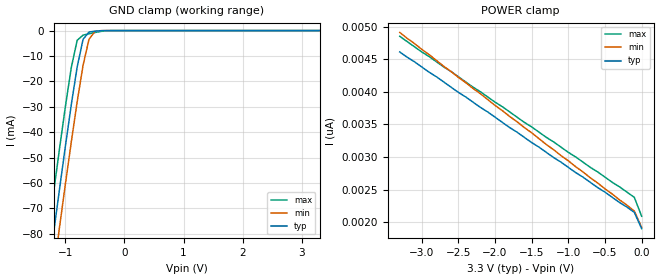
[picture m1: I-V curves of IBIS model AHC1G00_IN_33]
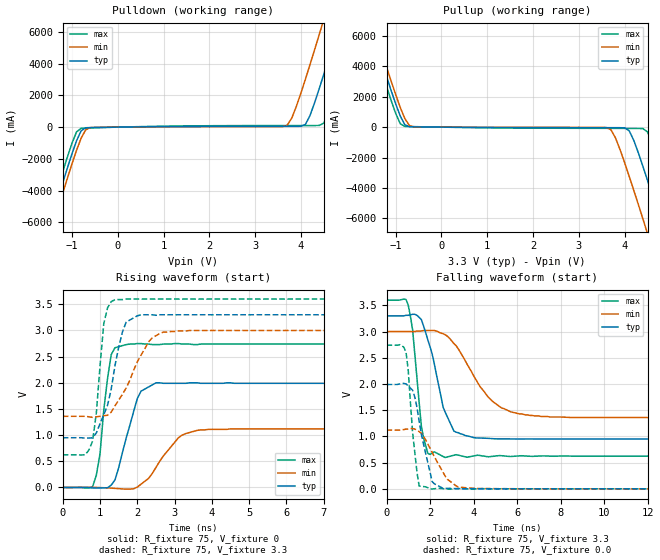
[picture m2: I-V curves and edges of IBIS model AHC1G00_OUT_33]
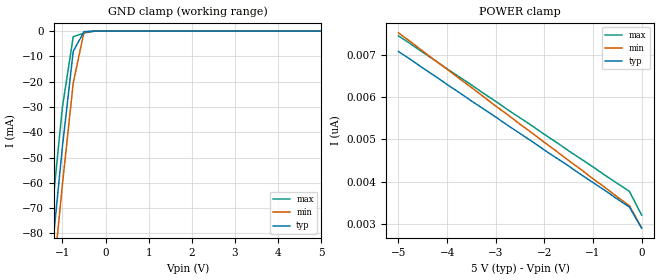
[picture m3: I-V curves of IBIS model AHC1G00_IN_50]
| TEXAS INSTRUMENTS INCORPORATED
| Standard Linear and Logic Group
| IBIS Model of SN74AHC1G00
| SINGLE 2-INPUT POSITIVE-NAND GATE
| SOT 5-pin (DCK) and SOT 5-pin (DBV) Package
[IBIS Ver]   3.2
[Comment Char]  |_char
[File Name]   ahc1g00.ibs
[File Rev]   2.0 J_die
[Date]   May 24, 2000
[Source]   Data created from HSPICE simulations at TI-SLL.
[Notes]   The following is an IBIS list for the AHC1G00.
|   Please contact sllibis@ti.com with questions and
|   comments concerning SLL IBIS models.
[Disclaimer] Property of Texas Instruments Incorporated.  Unauthorized
   reproduction and/or distribution is strictly prohibited.
   This product is protected under copyright law.
   Created 2000, (C) Copyright 2000, Texas Instruments Inc.,
   All Rights Reserved.
   UNLESS THERE IS A SIGNED, WRITTEN AGREEMENT TO THE
   CONTRARY, TEXAS INSTRUMENTS () IS PROVIDING THE IBIS
   MODELS  AND WITHOUT ANY WARRANTY, EXPRESSED OR
   IMPLIED.  TI assumes no liability for:
   1) the accuracy of the IBIS models provided to your
   company;
   2) the proper functioning of these IBIS Models in your
   design or for any resulting applications; or
   3) infringement of patents, copyrights or intellectual
   property rights resulting from your use of these IBIS
   models.
   TI provides IBIS Models as a service to our customers.
   You and your company shall not distribute, sell or give
   these models to anyone else without prior written
   permission from TI.
   TI reserves the right to make changes to our products or
   to discontinue any semiconductor product or service
   without notice, and advises our customers to obtain the
   latest version of relevant information to verify, before
   placing orders, that the information being relied on is
   current.
   Please be aware that your receipt and use of the IBIS
   information provided shall serve as acceptance of these
   terms and conditions.  If you do not accept these terms,
   you should return or destroy the IBIS models and any
   other accompanying information immediately.
|   Component AHC1G00_DCK
[Component]   AHC1G00_DCK
[Manufacturer]  Texas Instruments, Inc.
[Package]
|   typ   min   max
R_pkg   0.020   0.017   0.025
L_pkg   0.998nH   0.881nH   1.069nH
C_pkg   0.146pF   0.118pF   0.205pF
[Pin]   signal_name   model_name   R_pin   L_pin   C_pin
1   A   AHC1G00_IN   0.019   1.069nH   0.162pF
2   B   AHC1G00_IN   0.018   0.881nH   0.121pF
3   GND   GND   0.017   1.031nH   0.205pF
4   Y   AHC1G00_OUT   0.020   0.960nH   0.124pF
5   VCC   POWER   0.025   1.049nH   0.118pF
|   Component AHC1G00_DBV
[Component]   AHC1G00_DBV
[Manufacturer]  Texas Instruments, Inc.
[Package]
|   typ   min   max
R_pkg   0.025   0.021   0.029
L_pkg   1.529nH   1.312nH   1.906nH
C_pkg   0.156pF   0.110pF   0.240pF
[Pin]   signal_name   model_name   R_pin   L_pin   C_pin
1   A   AHC1G00_IN   0.021   1.511nH   0.144pF
2   B   AHC1G00_IN   0.023   1.312nH   0.138pF
3   GND   GND   0.029   1.906nH   0.240pF
4   Y   AHC1G00_OUT   0.026   1.541nH   0.150pF
5   VCC   POWER   0.025   1.374nH   0.110pF
[Model Selector]   AHC1G00_IN
AHC1G00_IN_33   3.3-V Vcc Input Model
AHC1G00_IN_50   5.0-V Vcc Input Model
[Model Selector]   AHC1G00_OUT
AHC1G00_OUT_33   3.3-V Vcc Output Model
AHC1G00_OUT_50   5.0-V Vcc Output Model
| Models and submodels in the file (4): AHC1G00_IN_33 (Input), AHC1G00_OUT_33 (Output), AHC1G00_IN_50 (Input), AHC1G00_OUT_50 (Output)
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|   Model AHC1G00_IN_33
[Model]   AHC1G00_IN_33
Model_type  Input
Polarity   Inverting
Vinl = 0.99
Vinh = 2.31
| variable   typ   min   max
C_comp   1.27pf   0.95pf   1.59pf
[Temperature Range]   25   85   -40
[Voltage Range]   3.3   3.0   3.6
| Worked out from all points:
|   GND clamp passes 1 mA (typ) near -0.61 V on its own axis
[GND Clamp]
|   Voltage   I(typ)   I(min)   I(max)
-3.3V     -460mA     -475mA     -445mA
-1.3V     -97.5mA    -113mA     -81.5mA
-1.2V     -79.9mA    -95mA      -63.9mA
-1.1V     -62.6mA    -77.6mA    -46.7mA
-1V       -45.6mA    -60.5mA    -30mA
-900mV    -29.2mA    -43.9mA    -14.6mA
-800mV    -14.3mA    -28mA      -3.81mA
-700mV    -3.42mA    -13.6mA    -1.78mA
-600mV    -581uA     -3.4mA     -1.25mA
-500mV    -233uA     -353uA     -759uA
-400mV    -58.1uA    -21.9uA    -324uA
3.3V      1.9nA      2.34nA     1.69nA
[POWER Clamp]
|   Voltage   I(typ)   I(min)   I(max)
-3.3V     4.61nA     4.91nA     4.85nA
-3V       4.38nA     4.65nA     4.61nA
-100mV    2.15nA     2.17nA     2.38nA
0V        1.9nA      1.92nA     2.09nA
|   Model AHC1G00_OUT_33
[Model]   AHC1G00_OUT_33
Model_type  Output
Polarity   Inverting
Vmeas = 1.65v
Cref = 15pf
| variable   typ   min   max
C_comp   3.12pf   2.34pf   3.90pf
[Temperature Range]   25   85   -40
[Voltage Range]   3.3   3.0   3.6
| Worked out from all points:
|   slope of the pulldown table from 0 to 0.495 V, typ, clamps not added: 26.1 ohm
|   slope of the pullup table from 0 to 0.495 V, typ, clamps not added: 40.3 ohm
|   rising waveform, R_fixture 75, V_fixture 0: 20-80 % time 450ps typ, 685ps min, 249ps max; typ from 0 V to 1.99 V
|   falling waveform, R_fixture 75, V_fixture 3.3: 20-80 % time 837ps typ, 1.53ns min, 390ps max; typ from 3.3 V to 0.95 V
|   rising waveform, R_fixture 75, V_fixture 3.3: 20-80 % time 435ps typ, 701ps min, 222ps max; typ from 0.95 V to 3.3 V
|   falling waveform, R_fixture 75, V_fixture 0.0: 20-80 % time 576ps typ, 878ps min, 329ps max; typ from 1.99 V to 0 V
[Pulldown]
|   Voltage   I(typ)   I(min)   I(max)
-3.3V     -24A       -24.6A     -23.4A
-1.6V     -7.31A     -7.95A     -6.63A
-1.5V     -6.34A     -6.99A     -5.66A
-1V       -1.69A     -2.33A     -1.02A
-800mV    -234mA     -703mA     -70.7mA
-600mV    -28.4mA    -27.3mA    -48.1mA
3.7V      47.1mA     113mA      100mA
4.1V      173mA      3.03A      101mA
4.4V      2.42A      5.83A      105mA
4.8V      6.17A      9.67A      2.68A
5.2V      10A        13.6A      6.5A
6.6V      23.8A      27.4A      20.3A
[Pullup]
|   Voltage   I(typ)   I(min)   I(max)
-3.3V     23.8A      24.4A      23.2A
-1.6V     7.13A      7.74A      6.5A
-1.5V     6.17A      6.78A      5.53A
-1V       1.53A      2.14A      903mA
-800mV    158mA      559mA      49mA
-600mV    19.5mA     16.8mA     33.4mA
3.7V      -35.9mA    -168mA     -78.9mA
4.1V      -236mA     -3.23A     -83.5mA
4.4V      -2.58A     -6.03A     -95.5mA
4.8V      -6.34A     -9.88A     -2.81A
5.2V      -10.2A     -13.8A     -6.63A
6.6V      -24A       -27.6A     -20.4A
[Ramp]
| variable   typ   min   max
dV/dt_r   1.21E+00/4.52E-10   6.94E-01/6.99E-10   1.65E+00/2.52E-10
dV/dt_f   1.43E+00/7.64E-10   1.00E+00/1.55E-09   1.81E+00/3.63E-10
R_load = 75
[Rising Waveform]
R_fixture = 75
V_fixture = 0
|   Time   V(typ)   V(min)   V(max)
0s        0V         0V         0V
800ps     -8.66mV    1.87mV     14.2mV
1ns       -9.36mV    -2.54mV    650mV
1.1ns     -7.48mV    -5.53mV    1.48V
1.3ns     45.1mV     -12.5mV    2.54V
1.7ns     942mV      -32.5mV    2.73V
2.1ns     1.84V      63mV       2.75V
3.1ns     1.99V      948mV      2.75V
3.9ns     1.99V      1.11V      2.74V
25ns      1.99V      1.12V      2.74V
[Falling Waveform]
R_fixture = 75
V_fixture = 3.3
V_fixture_min = 3.0
V_fixture_max = 3.6
|   Time   V(typ)   V(min)   V(max)
0s        3.3V       3V         3.6V
1ns       3.31V      3V         3.5V
1.2ns     3.33V      3V         3.03V
1.6ns     3.23V      3.01V      1.2V
2ns       2.71V      3.02V      657mV
2.6ns     1.56V      2.96V      617mV
3.1ns     1.1V       2.77V      641mV
4ns       978mV      2.16V      626mV
6.8ns     950mV      1.39V      621mV
25ns      950mV      1.36V      624mV
[Rising Waveform]
R_fixture = 75
V_fixture = 3.3
V_fixture_min = 3.0
V_fixture_max = 3.6
|   Time   V(typ)   V(min)   V(max)
0s        950mV      1.36V      624mV
600ps     944mV      1.36V      624mV
800ps     950mV      1.34V      886mV
900ps     1.04V      1.35V      1.42V
1.1ns     1.39V      1.37V      3.13V
1.4ns     2.33V      1.56V      3.59V
1.7ns     3.16V      1.9V       3.6V
2.3ns     3.3V       2.78V      3.6V
2.7ns     3.3V       2.97V      3.6V
25ns      3.3V       3V         3.6V
[Falling Waveform]
R_fixture = 75
V_fixture = 0.0
|   Time   V(typ)   V(min)   V(max)
0s        1.99V      1.12V      2.74V
900ps     2V         1.14V      2.6V
1ns       1.96V      1.14V      2.25V
1.2ns     1.88V      1.15V      1.07V
1.5ns     1.29V      1.09V      53.9mV
2ns       317mV      775mV      -3.03mV
2.2ns     95.8mV     613mV      1.32mV
2.8ns     8.4mV      181mV      -4.28mV
3.7ns     1.56mV     18.6mV     -914uV
25ns      0V         0V         0V
|   Model AHC1G00_IN_50
[Model]   AHC1G00_IN_50
Model_type  Input
Polarity   Inverting
Vinl = 1.5
Vinh = 3.5
| variable   typ   min   max
C_comp   1.27pf   0.95pf   1.59pf
[Temperature Range]   25   85   -40
[Voltage Range]   5.0   4.5   5.5
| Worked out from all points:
|   GND clamp passes 1 mA (typ) near -0.52 V on its own axis
[GND Clamp]
|   Voltage   I(typ)   I(min)   I(max)
-5V       -773mA     -786mA     -758mA
-1.5V     -133mA     -148mA     -117mA
-1.25V    -88.7mA    -104mA     -72.7mA
-1V       -45.6mA    -60.5mA    -30mA
-750mV    -7.99mA    -20.5mA    -2.23mA
-500mV    -233uA     -353uA     -759uA
-250mV    -2.63nA    -182nA     -26.9uA
5V        2.9nA      3.64nA     2.54nA
[POWER Clamp]
|   Voltage   I(typ)   I(min)   I(max)
-5V       7.08nA     7.52nA     7.45nA
-1.5V     4.37nA     4.5nA      4.73nA
-250mV    3.4nA      3.43nA     3.77nA
0V        2.9nA      2.91nA     3.21nA
